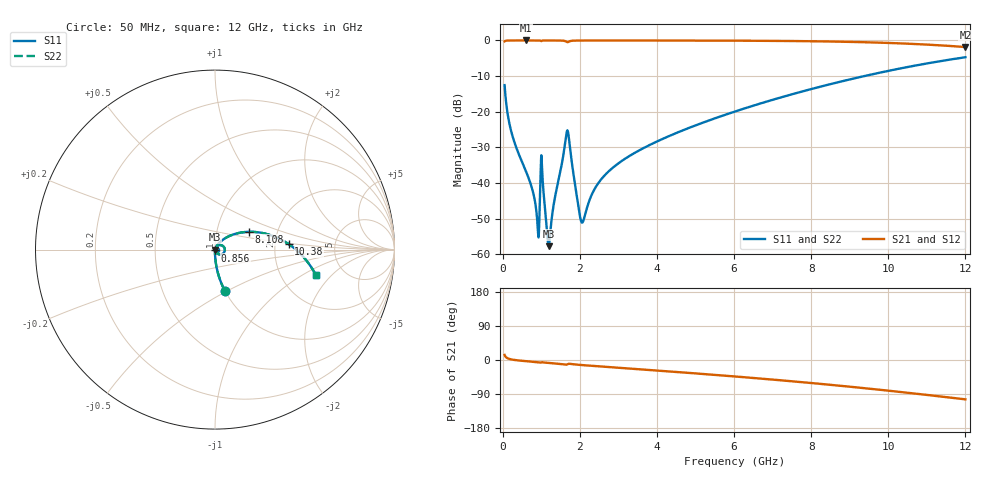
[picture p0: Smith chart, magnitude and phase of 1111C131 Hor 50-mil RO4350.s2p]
# GHz S MA R 50
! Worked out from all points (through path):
!   11951 points, 50 MHz to 12 GHz, reference 50 ohm
!   highest |S21| = -0.01 dB at 597 MHz (marker M1); lowest = -1.9 dB at 12 GHz (marker M2)
!   group delay of S21, straight-line fit = 23.9 ps
!   lowest |S11| = -57.7 dB at 1.191 GHz (marker M3), VSWR 1.00, Z = 50.1 - j0.0196 ohm
!   |S11| at or under -10 dB: start of sweep to 9.377 GHz
!   |S22| runs from -57.7 to -4.7 dB; largest |S21 - S12| = 0
!   S11 on the Smith chart (normalised r, x): 50 MHz: 1.00, -0.49; 856 MHz: 1.00, -0.01; 8.108 GHz: 1.44, +0.30; 10.38 GHz: 2.39, +0.17; 12 GHz: 3.13, -1.36
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0.05  0.2362 -76.6  0.9714 13.3  0.9714 13.3  0.2362 -76.6
0.236  0.04951 -88.2  0.9983 1.3  0.9983 1.3  0.04951 -88.2
0.597  0.01492 -90.3  0.9992 -3.0  0.9992 -3.0  0.01492 -90.3
0.856  0.004784 -83.3  0.9989 -5.3  0.9989 -5.3  0.004784 -83.3
0.916  0.002057 -52.3  0.9985 -5.9  0.9985 -5.9  0.002057 -52.3
0.999  0.02403 -7.7  0.9759 -6.5  0.9759 -6.5  0.02403 -7.7
1.029  0.01304 -70.1  0.9942 -6.0  0.9942 -6.0  0.01304 -70.1
1.143  0.002308 -61.8  0.9986 -7.3  0.9986 -7.3  0.002308 -61.8
1.191  0.001303 -8.6  0.9986 -7.7  0.9986 -7.7  0.001303 -8.6
1.671  0.05434 5.4  0.9479 -11.8  0.9479 -11.8  0.05434 5.4
1.721  0.04125 -41.0  0.9643 -10.0  0.9643 -10.0  0.04125 -41.0
1.951  0.005174 -55.7  0.9961 -12.5  0.9961 -12.5  0.005174 -55.7
2.042  0.002846 -14.1  0.997 -13.2  0.997 -13.2  0.002846 -14.1
2.37  0.008004 60.2  0.9979 -15.8  0.9979 -15.8  0.008004 60.2
2.676  0.01337 64.3  0.998 -18.0  0.998 -18.0  0.01337 64.3
4.034  0.03902 59.2  0.9971 -28.0  0.9971 -28.0  0.03902 59.2
6.025  0.1008 45.1  0.9921 -43.5  0.9921 -43.5  0.1008 45.1
8.017  0.2091 28.2  0.9742 -60.9  0.9742 -60.9  0.2091 28.2
8.108  0.2154 27.4  0.9728 -61.7  0.9728 -61.7  0.2154 27.4
10.009  0.3749 8.3  0.9222 -81.0  0.9222 -81.0  0.3749 8.3
10.385  0.4121 4.2  0.9061 -85.2  0.9061 -85.2  0.4121 4.2
12  0.5811 -14.3  0.8077 -103.8  0.8077 -103.8  0.5811 -14.3
